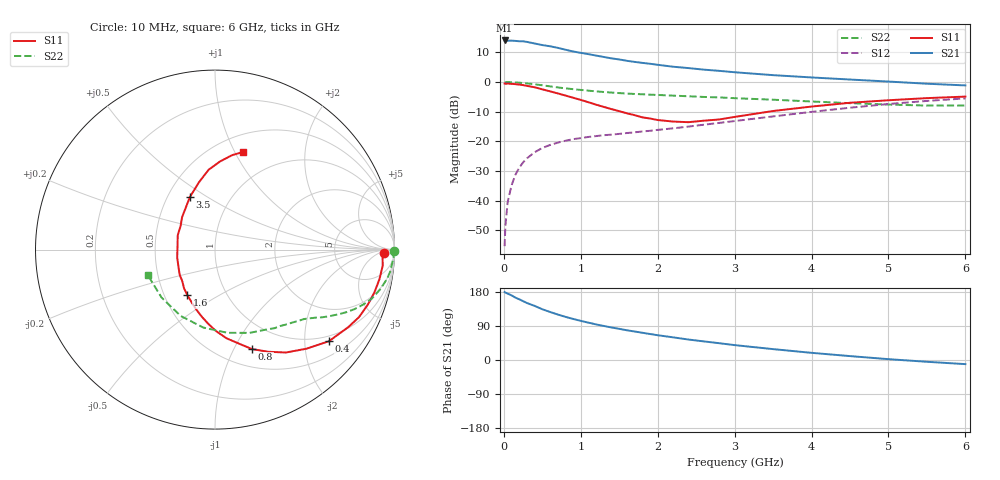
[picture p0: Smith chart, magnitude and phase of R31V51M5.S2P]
! SIEMENS Small Signal Semiconductors
! BFR181
! Si NPN RF Bipolar Junction Transistor in SOT23
! VCE = 1.5 V  IC = 1.5 mA
! Common Emitter S-Parameters:  May  1996
# GHz  S  MA  R  50
!  f  S11  S21  S12  S22
! GHz  MAG  ANG  MAG  ANG  MAG  ANG  MAG  ANG
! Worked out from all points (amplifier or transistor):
!   36 points, 10 MHz to 6 GHz, reference 50 ohm
!   highest |S21| = 14.0 dB at 10 MHz (marker M1)
!   |S21| within 3 dB of that: start of sweep to 782.1 MHz
!   unconditionally stable (mu >= 1): 1.699 GHz to 3.569 GHz
!   at 250 MHz: K = 0.20, MSG = 20.4 dB, |S12| = -27.1 dB
!   at 1.4 GHz: K = 0.89, MSG = 12.9 dB, |S12| = -17.8 dB
!   at 6 GHz: K = 0.88, MSG = 2.2 dB, |S12| = -5.5 dB
!   S11 on the Smith chart (normalised r, x): 10 MHz: 31, -9; 400 MHz: 0.85, -2.59; 800 MHz: 0.69, -1.18; 1.6 GHz: 0.65, -0.36; 3.5 GHz: 0.65, +0.42; 6 GHz: 0.67, +1.08
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0.01  0.9418 -1.0  5.018 179.3  0.0017 90.0  0.9982 -0.5
0.02  0.9339 -2.0  5.013 177.9  0.0037 84.3  0.9909 -1.0
0.05  0.9388 -5.4  4.978 175.2  0.0095 86.7  0.9959 -2.4
0.1  0.931 -10.2  4.988 170.5  0.018 84.5  0.9895 -4.7
0.15  0.9194 -15.1  4.929 164.7  0.0272 79.6  0.983 -7.3
0.25  0.8862 -25.1  4.855 155.3  0.044 74.4  0.9596 -11.5
0.3  0.8595 -30.1  4.745 150.4  0.0515 71.9  0.9451 -13.7
0.4  0.8146 -38.8  4.462 142.8  0.0653 66.8  0.9151 -17.4
0.5  0.7514 -47.3  4.195 133.9  0.077 62.8  0.8803 -20.4
0.6  0.6964 -55.4  4.007 126.8  0.0865 59.2  0.8437 -23.2
0.8  0.5912 -69.6  3.507 113.9  0.1019 53.6  0.7818 -27.3
0.9  0.5435 -75.3  3.271 108.4  0.1086 51.9  0.7568 -28.9
1.1  0.4552 -89.1  2.948 98.6  0.1183 49.6  0.7133 -31.8
1.3  0.38 -101.3  2.641 89.8  0.1266 48.3  0.6772 -34.0
1.6  0.2961 -121.5  2.275 78.4  0.1377 48.4  0.6383 -37.1
1.9  0.2421 -144.2  2.03 68.6  0.1502 49.4  0.6111 -40.4
2.2  0.215 -168.5  1.809 59.8  0.1653 50.6  0.5886 -44.0
2.8  0.2333 145.1  1.541 44.3  0.2041 52.1  0.5491 -52.9
3.5  0.3238 115.7  1.304 28.7  0.2626 51.1  0.5025 -67.4
4.5  0.4461 94.6  1.1 10.3  0.3681 44.0  0.4392 -98.5
5.5  0.5343 79.8  0.935 -4.7  0.4793 31.4  0.4 -138.1
6  0.5671 73.8  0.875 -10.9  0.5285 24.0  0.4003 -159.0
